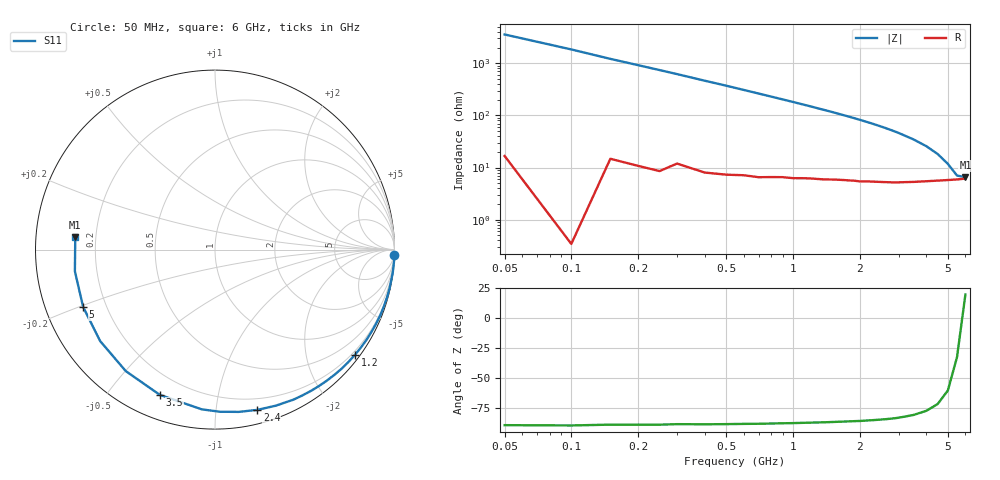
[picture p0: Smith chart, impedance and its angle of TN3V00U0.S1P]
! SIEMENS Discrete & RF Semiconductors
! BAS70-07W
! Si Schottky Diode in SOT343
! VR = 3 V
! S-Parameters:  February  1997
# GHz  S  MA  R  50
!  f  S11
! GHz  MAG  ANG
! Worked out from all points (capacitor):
!   34 points, 50 MHz to 6 GHz, reference 50 ohm
!   read as one part to ground: C = 870 fF near 50 MHz
!   lowest |Z| = 6.52 ohm at 6 GHz (marker M1)
!   series resonance near 5.817 GHz, so ESL is about 860 pH
!   S11 on the Smith chart (normalised r, x): 50 MHz: 0, -72; 1.2 GHz: 0.12, -2.98; 2.4 GHz: 0.11, -1.29; 3.5 GHz: 0.11, -0.68; 5 GHz: 0.12, -0.21; 6 GHz: 0.12, +0.04
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0.05  0.9999 -1.6
0.1  1 -3.1
0.25  0.9985 -7.7
0.4  0.9963 -12.3
0.5  0.9948 -15.3
0.6  0.9928 -18.4
0.7  0.991 -21.5
0.8  0.9882 -24.6
1  0.9825 -30.8
1.2  0.9754 -37.0
1.3  0.9719 -40.2
1.4  0.9684 -43.3
1.5  0.964 -46.4
1.6  0.9597 -49.6
1.7  0.9554 -52.8
1.8  0.9514 -55.9
2  0.9435 -62.3
2.2  0.9333 -68.7
2.4  0.9236 -75.2
2.6  0.9138 -81.7
2.8  0.9039 -88.2
3  0.8932 -94.7
3.5  0.8657 -110.8
4  0.8399 -126.3
4.5  0.818 -141.5
5  0.8012 -156.5
5.5  0.7899 -171.2
6  0.7817 174.9
